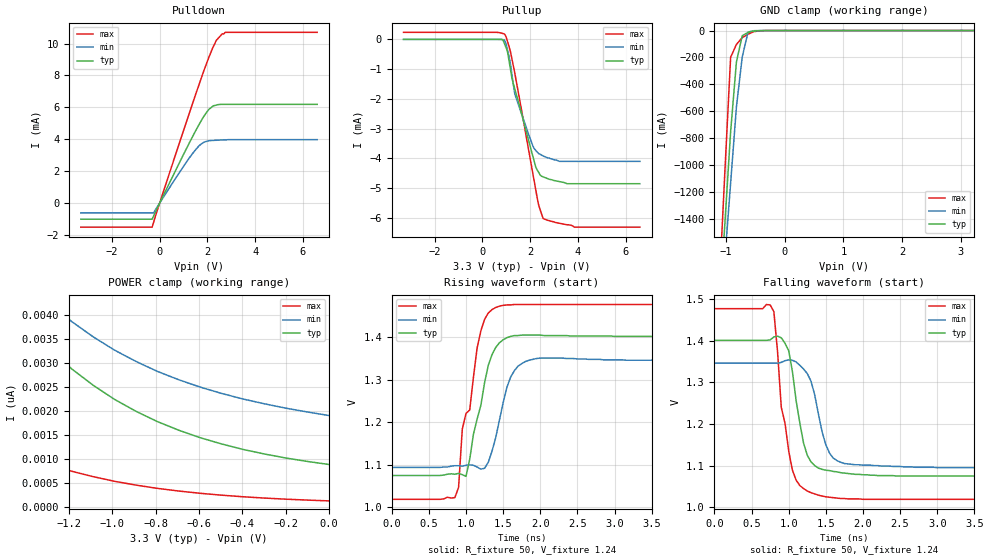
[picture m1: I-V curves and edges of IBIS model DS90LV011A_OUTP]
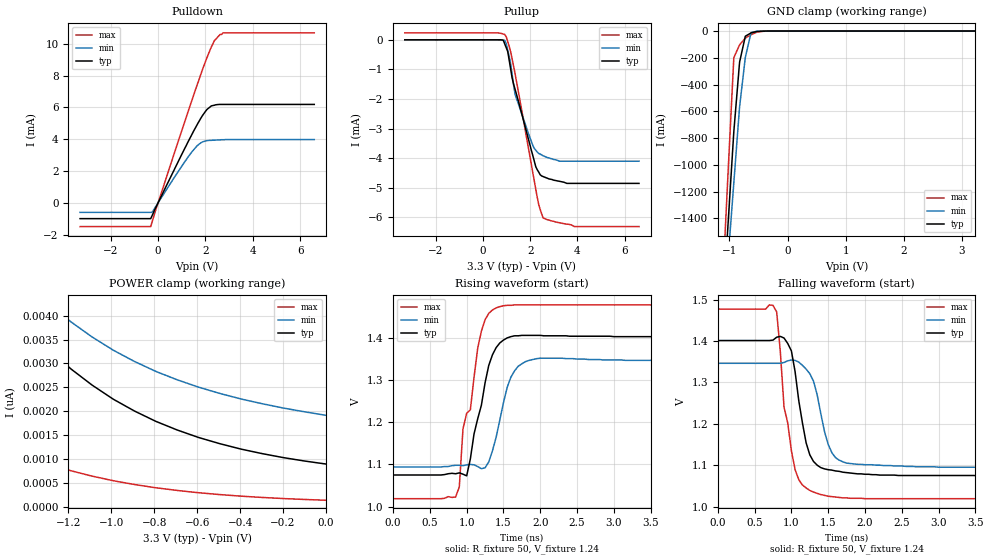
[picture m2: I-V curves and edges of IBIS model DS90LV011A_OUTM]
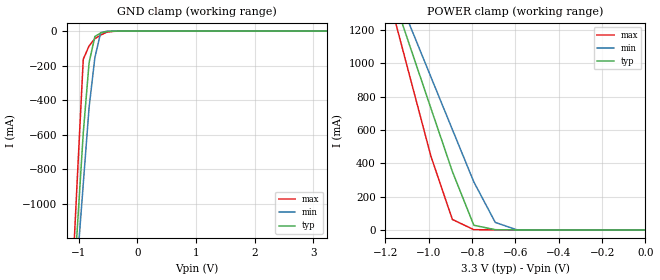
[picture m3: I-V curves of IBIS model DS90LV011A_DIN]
|   National Semiconductor Corporation
|   IBIS Model of DS90LV011A
|   3V LVDS Single High Speed Differential Driver
|   8 Lead LLP Package
[IBIS Ver]   3.2
[Comment Char]   |_char
[File name]   ds90lv011atld.ibs
[File Rev]   1.0
[Date]   10/3/02
[Source]
SPICE to IBIS Translation
[Notes]
* Rev 1.0 Comments:
Parser Results:
Checking ds90lv011atld.ibs for IBIS 3.2 Compatibility...
Errors  : 0
File Passed
Model Comments:
Created By: Tim Coyle
* END Rev 1.0 Comments
[Disclaimer]
(C) Copyright National Semiconductor Corporation 2002
   All rights reserved
   National Semiconductor Corporation hereby grants
the user of this IBIS model a non-exclusive, nontransferable
license to use this IBIS model under the following terms.
Before using this IBIS model, the user should read this
license.  If the user does not accept these terms,  the
IBIS model should be returned to National within 30 days.
   The user is granted this license only to use the
IBIS model and is not granted rights to sell, load, rent,
lease or license the IBIS model in whole or in part, or in
modified form to anyone other than user. User may modify
the IBIS model to suit its specific applications but rights
to derivative works and such modifications shall belong to
National.
   This IBIS model is provided on an "AS IS" basis and
National makes absolutely no warranty with respect to the
information contained herein.NATIONAL DISCLAIMS AND CUSTOMER
WAIVES ALL WARRANTIES, EXPRESS OR IMPLIED, INCLUDING
WARRANTIES OF MERCHANTABILITY OR FITNESS FOR A PARTICULAR
PURPOSE. The entire risk as to quality and performance is
with the Customer. ACCORDINGLY, IN NO EVENT SHALL THE
COMPANY BE LIABLE FOR ANY DAMAGES, WHETHER IN CONTRACT OR
TORT,INCLUDING ANY LOST PROFITS OR OTHER INCIDENTAL,
CONSEQUENTIAL, EXEMPLARY, OR PUNITIVE DAMAGES ARISING OUT
OF THE USE OR APPLICATION OF THE IBIS model provided in
this package.Further, National reserves the right to make
changes without notice to any product herein to improve
reliability, function, or design. National does not convey
any license under patent rights or any other intellectual
property rights, including those of third parties.
   National is not obligated to provide maintenance or support
for the licensed IBIS model.
Contact National at ATTN:INTERFACE APPLICATIONS/IBIS MODELS.
5 Foden Road, M/S 03-03, South Porltand, ME 04106
(207) 541-8203
[Copyright]
(c) Copyright 2002 National Semiconductor Corp.
[Component]   DS90LV011A
Si_location Pin
Timing_location Pin
[Manufacturer]   National Semiconductor Corp.
[Package]
|   TYP   MIN   MAX
R_pkg   1.000m   NA   NA
L_pkg   0.008n   NA   NA
C_pkg   0.030p   NA   NA
[Pin]   signal_name   model_name   R_pin   L_pin   C_pin
1   out+   DS90LV011A_OUTP   1.000m  0.008n  0.030p
2   gnd   GND   1.000m  0.008n  0.030p
3   out-   DS90LV011A_OUTM   1.000m  0.008n  0.030p
4   nc   NC   1.000m  0.008n  0.030p
5   nc   NC   1.000m  0.008n  0.030p
6   vdd   POWER   1.000m  0.008n  0.030p
7   gnd   GND   1.000m  0.008n  0.030p
8   ttl_in   DS90LV011A_DIN   1.000m  0.008n  0.030p
[Diff Pin] inv_pin   vdiff   tdelay_typ   tdelay_min   tdelay_max
| The '+' pin is Diff_pin and the '-' pin is the inv_pin
| Receiver Vth = +/-30mV
3   1   0   0   0   0
| Models and submodels in the file (3): DS90LV011A_OUTP (3-state), DS90LV011A_OUTM (3-state), DS90LV011A_DIN (Input)
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[Model]   DS90LV011A_OUTP
Model_type 3-state
Enable Active-High
Polarity Non-Inverting
Vref=1.21
Vmeas=1.21
Rref=50   | 100 Ohms Across Outputs OUTP and OUTM
Cref=15p
| Cref of 15p is total jig capacitance (distributed)
|   TYP   MIN   MAX
C_comp   4p   4p   4p
[Temperature Range] 25   85   -40
[Voltage Range]   3.30   3.00   3.60
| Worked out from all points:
|   slope of the pulldown table from 0 to 0.495 V, typ, clamps not added: 327 ohm
|   GND clamp passes 1 mA (typ) near -0.42 V on its own axis
|   falling waveform, R_fixture 50, V_fixture 1.24: 20-80 % time 184ps typ, 203ps min, 183ps max; typ from 1.4 V to 1.07 V
|   rising waveform, R_fixture 50, V_fixture 1.24: 20-80 % time 231ps typ, 209ps min, 240ps max; typ from 1.07 V to 1.4 V
[Pullup]
|Vtable   I(typ)   I(min)   I(max)
-3.3V     1.3nA      2.13nA     237uA
800mV     -1.95uA    -4.2uA     212uA
925mV     -138uA     -16uA      182uA
1.112V    -680uA     -547uA     -215uA
1.238V    -1.29mA    -1.17mA    -646uA
1.362V    -1.67mA    -1.84mA    -1.14mA
2.112V    -3.91mA    -3.57mA    -4.49mA
2.238V    -4.29mA    -3.73mA    -5.05mA
2.362V    -4.47mA    -3.84mA    -5.57mA
2.55V     -4.62mA    -3.92mA    -6.02mA
3.862V    -4.85mA    -4.1mA     -6.31mA
6.6V      -4.85mA    -4.1mA     -6.31mA
[Pulldown]
|V(pulldown)   I(typ)   I(min)   I(max)
-3.3V     -1mA       -603uA     -1.5mA
-313mV    -1mA       -603uA     -1.5mA
-250mV    -796uA     -603uA     -1.19mA
875mV     2.67mA     2.03mA     3.98mA
1.625V    4.85mA     3.55mA     7.31mA
1.812V    5.34mA     3.78mA     8.12mA
2V        5.75mA     3.89mA     8.88mA
2.25V     6.1mA      3.93mA     9.81mA
2.375V    6.14mA     3.94mA     10.2mA
2.625V    6.19mA     3.96mA     10.6mA
2.75V     6.19mA     3.97mA     10.7mA
6.6V      6.19mA     3.98mA     10.7mA
[GND Clamp]
|V(groundclamp)   I(typ)   I(min)   I(max)
-3.3V     -17.79A    -15.11A    -22.31A
-1.122V   -2.13A     -2.273A    -1.936A
-1.023V   -1.44A     -1.703A    -1.057A
-924mV    -751.6mA   -1.134A    -198.9mA
-825mV    -232.9mA   -567.3mA   -103.3mA
-726mV    -38.72mA   -196.7mA   -52.72mA
-627mV    -13.96mA   -11.49mA   -27.64mA
-528mV    -3.584mA   -1.412mA   -8.348mA
-330mV    -123.4uA   -52.37uA   -268.9uA
3.234V    857.1pA    2.099nA    93.12pA
[POWER Clamp]
|V(table)   I(typ)   I(min)   I(max)
-3.267V   46.62nA    40.29nA    20.01nA
-2.277V   12.92nA    12.82nA    4.536nA
-2.178V   11.26nA    11.38nA    3.87nA
-1.98V    8.554nA    9.002nA    2.81nA
-1.881V   7.457nA    8.027nA    2.393nA
-1.683V   5.654nA    6.409nA    1.724nA
-1.485V   4.298nA    5.176nA    1.239nA
-1.287V   3.289nA    4.247nA    889pA
-1.089V   2.545nA    3.553nA    639.8pA
-891mV    2.001nA    3.039nA    463.6pA
-495mV    1.32nA     2.372nA    253.7pA
0V        893pA      1.913nA    134.7pA
[Ramp]
|   TYP   MIN   MAX
dV/dt_r   196mV/.233ns   153mV/.244ns   276mV/.211ns
dV/dt_f   196mv/.190ns   153mV/.216ns   276mV/.180ns
R_load=50
[Falling Waveform]
R_fixture=50
V_fixture=1.24
V_fixture_min=1.22
V_fixture_max=1.25
|Time   V(typ)   V(min)   V(max)
0s        1.401V     1.346V     1.477V
800ps     1.409V     1.346V     1.47V
850ps     1.411V     1.346V     1.373V
900ps     1.407V     1.348V     1.24V
1ns       1.376V     1.354V     1.135V
1.1ns     1.256V     1.349V     1.065V
1.25ns    1.125V     1.321V     1.039V
1.5ns     1.089V     1.15V      1.025V
1.7ns     1.083V     1.108V     1.021V
4.95ns    1.075V     1.094V     1.019V
[Rising Waveform]
R_fixture=50
V_fixture=1.24
V_fixture_min=1.22
V_fixture_max=1.25
|Time   V(typ)   V(min)   V(max)
0s        1.075V     1.094V     1.019V
850ps     1.078V     1.098V     1.023V
900ps     1.08V      1.098V     1.047V
1ns       1.073V     1.099V     1.221V
1.05ns    1.113V     1.1V       1.229V
1.15ns    1.208V     1.095V     1.375V
1.4ns     1.376V     1.164V     1.47V
1.6ns     1.402V     1.306V     1.476V
1.85ns    1.405V     1.346V     1.477V
4.95ns    1.401V     1.346V     1.477V
[Model]   DS90LV011A_OUTM
Model_type 3-state
Enable Active-High
Polarity Inverting
Vref=1.21
Vmeas=1.21
Rref=50   | 100 Ohms Across Outputs OUTP and OUTM
Cref=15p
| Cref of 15p is total jig capacitance (distributed)
|   TYP   MIN   MAX
C_comp   4p   4p   4p
[Temperature Range] 25   85   -40
[Voltage Range]   3.30   3.00   3.60
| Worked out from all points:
|   slope of the pulldown table from 0 to 0.495 V, typ, clamps not added: 327 ohm
|   GND clamp passes 1 mA (typ) near -0.42 V on its own axis
|   falling waveform, R_fixture 50, V_fixture 1.24: 20-80 % time 184ps typ, 203ps min, 183ps max; typ from 1.4 V to 1.07 V
|   rising waveform, R_fixture 50, V_fixture 1.24: 20-80 % time 231ps typ, 209ps min, 240ps max; typ from 1.07 V to 1.4 V
[Pullup]
|Vtable   I(typ)   I(min)   I(max)
-3.3V     1.3nA      2.13nA     237uA
800mV     -1.95uA    -4.2uA     212uA
925mV     -138uA     -16uA      182uA
1.112V    -680uA     -547uA     -215uA
1.238V    -1.29mA    -1.17mA    -646uA
1.362V    -1.67mA    -1.84mA    -1.14mA
2.112V    -3.91mA    -3.57mA    -4.49mA
2.238V    -4.29mA    -3.73mA    -5.05mA
2.362V    -4.47mA    -3.84mA    -5.57mA
2.55V     -4.62mA    -3.92mA    -6.02mA
3.862V    -4.85mA    -4.1mA     -6.31mA
6.6V      -4.85mA    -4.1mA     -6.31mA
[Pulldown]
|V(pulldown)   I(typ)   I(min)   I(max)
-3.3V     -1mA       -603uA     -1.5mA
-313mV    -1mA       -603uA     -1.5mA
-250mV    -796uA     -603uA     -1.19mA
875mV     2.67mA     2.03mA     3.98mA
1.625V    4.85mA     3.55mA     7.31mA
1.812V    5.34mA     3.78mA     8.12mA
2V        5.75mA     3.89mA     8.88mA
2.25V     6.1mA      3.93mA     9.81mA
2.375V    6.14mA     3.94mA     10.2mA
2.625V    6.19mA     3.96mA     10.6mA
2.75V     6.19mA     3.97mA     10.7mA
6.6V      6.19mA     3.98mA     10.7mA
[GND Clamp]
|V(groundclamp)   I(typ)   I(min)   I(max)
-3.3V     -17.79A    -15.11A    -22.31A
-1.122V   -2.13A     -2.273A    -1.936A
-1.023V   -1.44A     -1.703A    -1.057A
-924mV    -751.6mA   -1.134A    -198.9mA
-825mV    -232.9mA   -567.3mA   -103.3mA
-726mV    -38.72mA   -196.7mA   -52.72mA
-627mV    -13.96mA   -11.49mA   -27.64mA
-528mV    -3.584mA   -1.412mA   -8.348mA
-330mV    -123.4uA   -52.37uA   -268.9uA
3.234V    857.1pA    2.099nA    93.12pA
[POWER Clamp]
|V(table)   I(typ)   I(min)   I(max)
-3.267V   46.62nA    40.29nA    20.01nA
-2.277V   12.92nA    12.82nA    4.536nA
-2.178V   11.26nA    11.38nA    3.87nA
-1.98V    8.554nA    9.002nA    2.81nA
-1.881V   7.457nA    8.027nA    2.393nA
-1.683V   5.654nA    6.409nA    1.724nA
-1.485V   4.298nA    5.176nA    1.239nA
-1.287V   3.289nA    4.247nA    889pA
-1.089V   2.545nA    3.553nA    639.8pA
-891mV    2.001nA    3.039nA    463.6pA
-495mV    1.32nA     2.372nA    253.7pA
0V        893pA      1.913nA    134.7pA
[Ramp]
|   TYP   MIN   MAX
dV/dt_r   196mV/.233ns   153mV/.244ns   276mV/.211ns
dV/dt_f   196mv/.190ns   153mV/.216ns   276mV/.180ns
R_load=50
[Falling Waveform]
R_fixture=50
V_fixture=1.24
V_fixture_min=1.22
V_fixture_max=1.25
|Time   V(typ)   V(min)   V(max)
0s        1.401V     1.346V     1.477V
800ps     1.409V     1.346V     1.47V
850ps     1.411V     1.346V     1.373V
900ps     1.407V     1.348V     1.24V
1ns       1.376V     1.354V     1.135V
1.1ns     1.256V     1.349V     1.065V
1.25ns    1.125V     1.321V     1.039V
1.5ns     1.089V     1.15V      1.025V
1.7ns     1.083V     1.108V     1.021V
4.95ns    1.075V     1.094V     1.019V
[Rising Waveform]
R_fixture=50
V_fixture=1.24
V_fixture_min=1.22
V_fixture_max=1.25
|Time   V(typ)   V(min)   V(max)
0s        1.075V     1.094V     1.019V
850ps     1.078V     1.098V     1.023V
900ps     1.08V      1.098V     1.047V
1ns       1.073V     1.099V     1.221V
1.05ns    1.113V     1.1V       1.229V
1.15ns    1.208V     1.095V     1.375V
1.4ns     1.376V     1.164V     1.47V
1.6ns     1.402V     1.306V     1.476V
1.85ns    1.405V     1.346V     1.477V
4.95ns    1.401V     1.346V     1.477V
[Model]   DS90LV011A_DIN
Model_type Input
Vinh=2.0
Vinl=0.8
|   TYP   MIN   MAX
C_comp   3p   3p   3p
[Temperature Range] 25   85   -40
[Voltage Range]   3.30   3.00   3.60
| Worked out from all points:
|   GND clamp passes 1 mA (typ) near -0.44 V on its own axis
|   POWER clamp passes 1 mA (typ) near -0.65 V on its own axis
[GND Clamp]
|V(groundclamp)   I(typ)   I(min)   I(max)
-3.3V     -13.98A    -11.83A    -17.63A
-1.122V   -1.669A    -1.777A    -1.526A
-1.023V   -1.129A    -1.331A    -837mA
-924mV    -590.8mA   -886.6mA   -163.5mA
-825mV    -184mA     -443.7mA   -85.99mA
-726mV    -31.28mA   -153.9mA   -44.23mA
-627mV    -11.3mA    -9.068mA   -22.94mA
-528mV    -2.886mA   -1.123mA   -6.914mA
-330mV    -102.6uA   -43.64uA   -229.3uA
3.234V    1.855uA    1.074uA    3.371uA
[POWER Clamp]
|V(table)   I(typ)   I(min)   I(max)
-3.267V   9.584A     8.291A     11.75A
-1.188V   1.491A     1.55A      1.416A
-1.089V   1.11A      1.233A     928.2mA
-990mV    729.5mA    917.3mA    441.9mA
-891mV    350.5mA    602.3mA    63.05mA
-792mV    28.24mA    288.1mA    1.817mA
-693mV    1.617mA    45.27mA    453.5uA
-594mV    118.9uA    1.221mA    66.77uA
0V        857.1pA    1.83nA     132.3pA
